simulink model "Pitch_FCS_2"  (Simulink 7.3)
settings: Solver=ode45  StartTime=0.0  StopTime=10.0  RelTol=1e-3

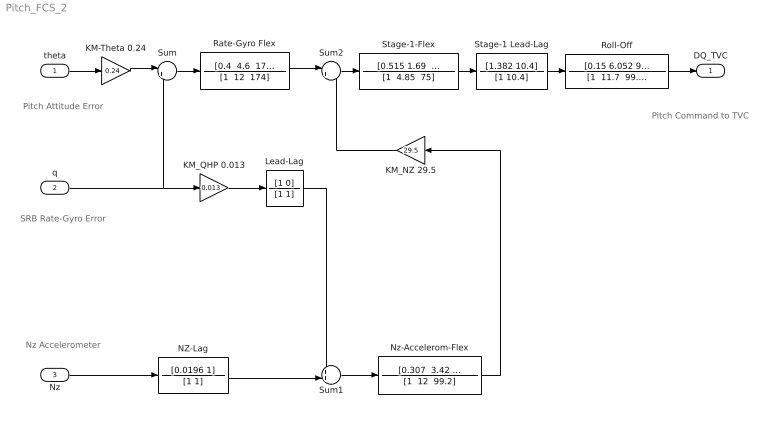
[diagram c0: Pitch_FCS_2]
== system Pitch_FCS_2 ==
  note: Nz Accelerometer
  note: Pitch Attitude Error
  note: SRB Rate-Gyro Error
  note: Pitch Command to TVC
  theta : Inport  OutDataType=fixdt(1, 16)  OutScaling=2^0
  q : Inport  Port=2  OutDataType=fixdt(1, 16)  OutScaling=2^0
  Nz : Inport  Port=3  OutDataType=fixdt(1, 16)  OutScaling=2^0
  KM-Theta 0.24 : Gain  Gain=0.24  ParameterDataType=fixdt(1, 16)  ParameterScaling=2^0  OutDataType=fixdt(1, 16)  OutScaling=2^0
  KM_NZ 29.5 : Gain  Gain=29.5  ParameterDataType=fixdt(1, 16)  ParameterScaling=2^0  OutDataType=fixdt(1, 16)  OutScaling=2^0
  KM_QHP 0.013 : Gain  Gain=0.013  ParameterDataType=fixdt(1, 16)  ParameterScaling=2^0  OutDataType=fixdt(1, 16)  OutScaling=2^0
  Lead-Lag : TransferFcn  Numerator=[1 0]  Denominator=[1 1]
  NZ-Lag : TransferFcn  Numerator=[0.0196 1]  Denominator=[1 1]
  Nz-Accelerom-Flex : TransferFcn  Numerator="[0.307  3.42  99.2]"  Denominator="[1  12  99.2]"
  Rate-Gyro Flex : TransferFcn  Numerator="[0.4  4.6  174]"  Denominator="[1  12  174]"
  Roll-Off : TransferFcn  Numerator=[0.15 6.052 99.2]  Denominator="[1  11.7  99.2]"
  Stage-1 Lead-Lag : TransferFcn  Numerator=[1.382 10.4]  Denominator=[1 10.4]
  Stage-1-Flex : TransferFcn  Numerator="[0.515 1.69  75]"  Denominator="[1  4.85  75]"
  Sum : Sum  Inputs=|++  OutDataType=fixdt(1, 16)  OutScaling=2^0
  Sum1 : Sum  Inputs=++|  OutDataType=fixdt(1, 16)  OutScaling=2^0
  Sum2 : Sum  Inputs=|++  OutDataType=fixdt(1, 16)  OutScaling=2^0
  DQ_TVC : Outport  OutDataType=fixdt(1, 16)  OutScaling=2^0
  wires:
  theta/1 -> KM-Theta 0.24/1
  KM-Theta 0.24/1 -> Sum/1
  Sum/1 -> Rate-Gyro Flex/1
  q/1 -> Sum/2, KM_QHP 0.013/1
  KM_QHP 0.013/1 -> Lead-Lag/1
  Nz/1 -> NZ-Lag/1
  Stage-1 Lead-Lag/1 -> Roll-Off/1
  Stage-1-Flex/1 -> Stage-1 Lead-Lag/1
  NZ-Lag/1 -> Sum1/2
  Sum1/1 -> Nz-Accelerom-Flex/1
  Lead-Lag/1 -> Sum1/1
  Rate-Gyro Flex/1 -> Sum2/1
  Sum2/1 -> Stage-1-Flex/1
  Nz-Accelerom-Flex/1 -> KM_NZ 29.5/1
  KM_NZ 29.5/1 -> Sum2/2
  Roll-Off/1 -> DQ_TVC/1
